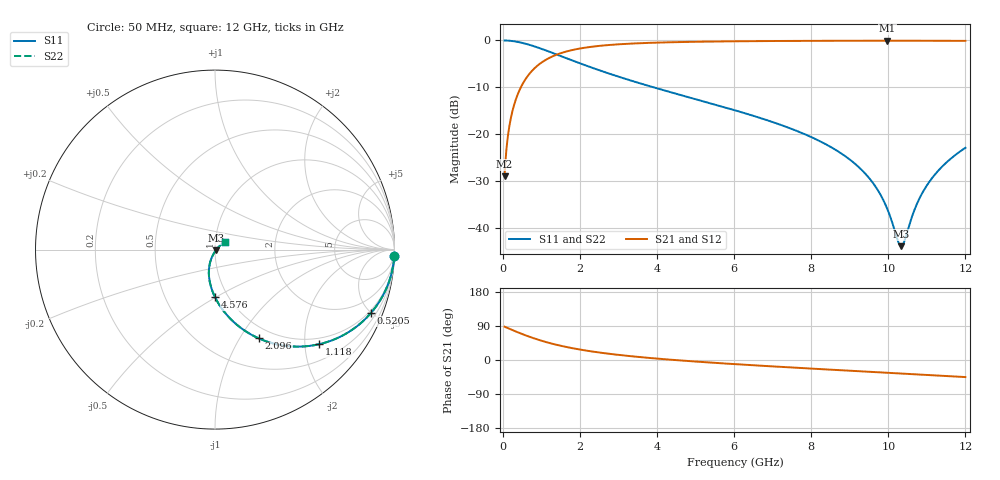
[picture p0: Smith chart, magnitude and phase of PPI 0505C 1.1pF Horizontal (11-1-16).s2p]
# MHz S MA R 50
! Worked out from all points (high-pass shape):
!   1601 points, 50 MHz to 12 GHz, reference 50 ohm
!   highest |S21| = -0.06 dB at 9.976 GHz (marker M1); lowest = -29.1 dB at 50 MHz (marker M2)
!   |S21| within 3 dB of the highest: 1.393 GHz to end of sweep
!   lowest |S11| = -44.0 dB at 10.33 GHz (marker M3), VSWR 1.01, Z = 50.5 - j0.38 ohm
!   |S11| at or under -10 dB: 3.902 GHz to end of sweep
!   |S22| runs from -44.0 to 0.0 dB; largest |S21 - S12| = 0
!   S11 on the Smith chart (normalised r, x): 50 MHz: 1, -52; 520.5 MHz: 0.85, -5.00; 1.118 GHz: 0.85, -2.31; 2.096 GHz: 0.85, -1.21; 4.576 GHz: 0.87, -0.49; 12 GHz: 1.11, +0.10
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50  0.9994 -2.2  0.03524 87.8  0.03524 87.8  0.9994 -2.2
147.0938  0.9946 -6.4  0.1032 83.5  0.1032 83.5  0.9946 -6.4
229.25  0.9871 -10.0  0.1596 80.0  0.1596 80.0  0.9871 -10.0
520.5312  0.9384 -22.0  0.3449 67.9  0.3449 67.9  0.9384 -22.0
1118.031  0.7828 -42.4  0.6207 47.5  0.6207 47.5  0.7828 -42.4
2044.156  0.5612 -62.9  0.8252 26.8  0.8252 26.8  0.5612 -62.9
2096.438  0.5511 -63.8  0.8319 26.0  0.8319 26.0  0.5511 -63.8
2932.938  0.419 -75.3  0.9049 14.3  0.9049 14.3  0.419 -75.3
4038.312  0.3046 -86.0  0.9488 3.4  0.9488 3.4  0.3046 -86.0
4576.062  0.2637 -90.1  0.9606 -0.9  0.9606 -0.9  0.2637 -90.1
6025  0.1792 -99.6  0.9791 -10.9  0.9791 -10.9  0.1792 -99.6
8019.156  0.09201 -109.5  0.9901 -22.8  0.9901 -22.8  0.09201 -109.5
9266.438  0.04302 -112.0  0.9927 -29.7  0.9927 -29.7  0.04302 -112.0
9669.75  0.02738 -109.4  0.9931 -32.0  0.9931 -32.0  0.02738 -109.4
9975.969  0.01577 -100.8  0.9931 -33.7  0.9931 -33.7  0.01577 -100.8
10013.31  0.01442 -98.6  0.9931 -33.9  0.9931 -33.9  0.01442 -98.6
10334.47  0.006325 -36.5  0.993 -35.7  0.993 -35.7  0.006325 -36.5
10416.62  0.007149 -9.1  0.993 -36.1  0.993 -36.1  0.007149 -9.1
10737.78  0.01769 30.4  0.9927 -37.9  0.9927 -37.9  0.01769 30.4
11014.12  0.02877 37.1  0.9922 -39.5  0.9922 -39.5  0.02877 37.1
11454.78  0.0473 39.6  0.9913 -41.9  0.9913 -41.9  0.0473 39.6
12000  0.07124 39.1  0.9895 -45.1  0.9895 -45.1  0.07124 39.1
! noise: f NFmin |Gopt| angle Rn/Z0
50  0.0011  0.967  1.582  0.007546
1372  0.005838  0.7693  6.971  0.005136
2701  0.009198  0.7178  11.25  0.006387
4031  0.01217  0.688  15.63  0.007445
5360  0.01496  0.6685  20  0.00842
6682  0.01767  0.6557  24.29  0.009368
8012  0.02038  0.6477  28.52  0.01034
9341  0.02314  0.6436  32.65  0.01136
1.067e+04  0.02599  0.6428  36.68  0.01246
1.2e+04  0.02897  0.6449  40.59  0.01368
